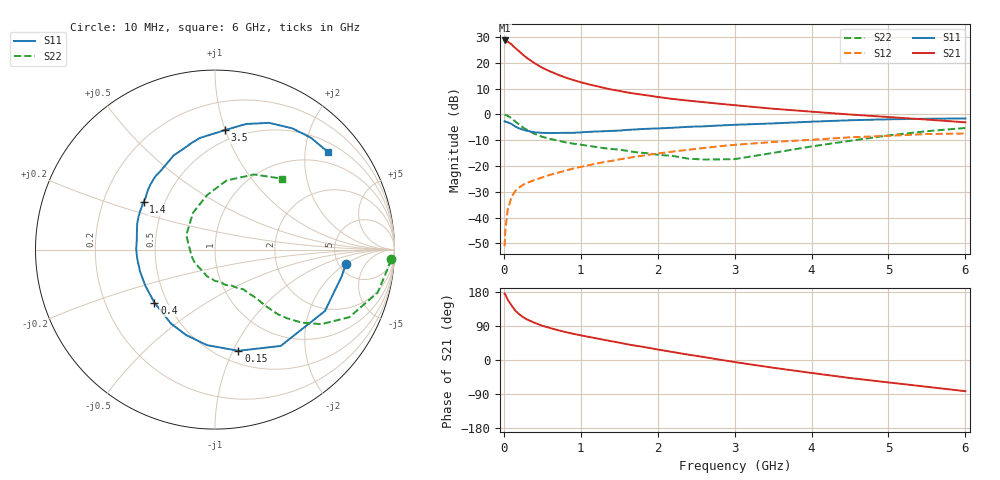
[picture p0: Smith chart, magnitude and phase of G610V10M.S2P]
! SIEMENS Small Signal Semiconductors
! BFG193
! Si NPN RF Bipolar Junction Transistor in SOT223
! VCE = 10 V  IC = 10 mA
! Common Emitter S-Parameters:  August  1996
# GHz  S  MA  R  50
!  f  S11  S21  S12  S22
! GHz  MAG  ANG  MAG  ANG  MAG  ANG  MAG  ANG
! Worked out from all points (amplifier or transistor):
!   36 points, 10 MHz to 6 GHz, reference 50 ohm
!   highest |S21| = 28.6 dB at 10 MHz (marker M1)
!   |S21| within 3 dB of that: start of sweep to 151.6 MHz
!   unconditionally stable (mu >= 1): 931.8 MHz to 2.534 GHz
!   at 250 MHz: K = 0.52, MSG = 25.2 dB, |S12| = -27.3 dB
!   at 1.4 GHz: K = 1.06, MAG = 12.3 dB, |S12| = -18.0 dB
!   at 6 GHz: K = 0.86, MSG = 2.2 dB, |S12| = -7.4 dB
!   S11 on the Smith chart (normalised r, x): 10 MHz: 5.83, -1.97; 150 MHz: 0.62, -1.05; 400 MHz: 0.43, -0.32; 1.4 GHz: 0.38, +0.26; 3.5 GHz: 0.41, +0.99; 6 GHz: 0.71, +2.51
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0.01  0.7336 -6.1  26.95 175.2  0.0028 88.4  0.9805 -3.1
0.02  0.7212 -12.0  26.64 172.1  0.0057 84.4  0.9692 -6.1
0.05  0.7016 -29.2  25.59 159.3  0.0141 76.4  0.9373 -14.8
0.1  0.6498 -55.7  22.64 144.0  0.0252 65.3  0.8376 -26.7
0.15  0.5786 -77.0  19.17 130.1  0.033 58.7  0.7241 -35.0
0.2  0.534 -94.9  16.52 120.8  0.0384 55.0  0.6338 -40.0
0.25  0.502 -108.8  14.18 113.0  0.0431 52.0  0.5554 -43.6
0.3  0.4799 -120.6  12.36 107.1  0.047 51.5  0.5023 -45.8
0.4  0.4488 -138.7  9.783 98.2  0.0535 50.2  0.4188 -48.2
0.5  0.4372 -152.8  7.986 90.3  0.06 50.2  0.3671 -49.3
0.6  0.435 -163.6  6.798 84.4  0.0673 50.9  0.3352 -50.6
0.7  0.4362 -173.1  5.886 78.9  0.0739 51.1  0.3094 -52.2
0.9  0.439 173.0  4.63 69.3  0.0892 50.7  0.271 -54.6
1.1  0.4573 161.4  3.823 61.2  0.1031 49.8  0.246 -60.1
1.4  0.4786 146.2  3.018 49.5  0.1255 46.9  0.2139 -68.5
1.7  0.5086 135.6  2.52 38.2  0.15 43.1  0.1858 -78.9
2.2  0.5505 118.9  1.981 20.9  0.1904 34.5  0.1564 -105.8
2.8  0.6076 102.5  1.606 1.1  0.2408 23.1  0.1343 -150.3
3.5  0.6672 85.4  1.283 -20.4  0.2914 7.4  0.1792 153.2
4.5  0.7679 66.9  0.992 -47.5  0.3589 -12.2  0.3072 98.2
5.5  0.821 49.3  0.791 -70.7  0.4161 -36.5  0.4715 62.6
6  0.8318 40.8  0.701 -82.3  0.4252 -50.6  0.544 46.6
